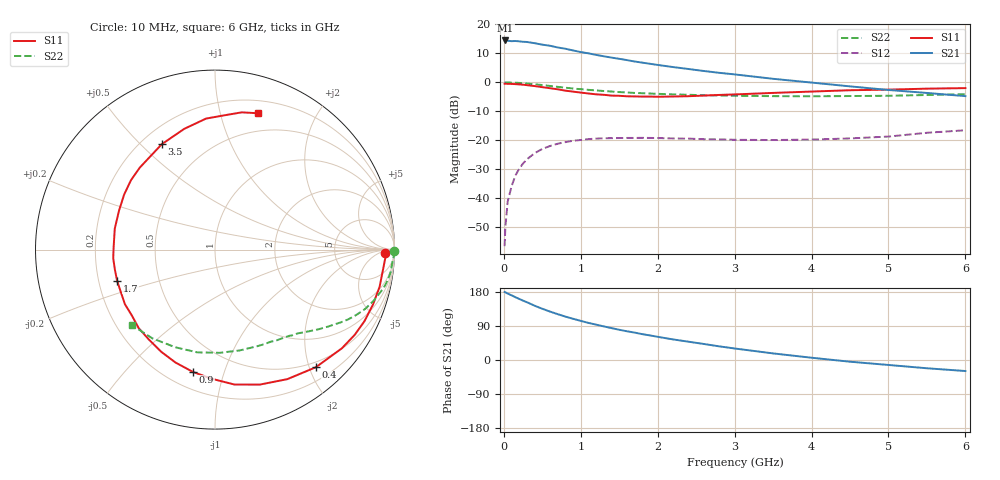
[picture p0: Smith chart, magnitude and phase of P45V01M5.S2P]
! SIEMENS Small Signal Semiconductors
! BFP182
! Si NPN RF Bipolar Junction Transistor in SOT143
! VCE = 5 V  IC = 1.5 mA
! Common Emitter S-Parameters:  March  1996
# GHz  S  MA  R  50
!  f  S11  S21  S12  S22
! GHz  MAG  ANG  MAG  ANG  MAG  ANG  MAG  ANG
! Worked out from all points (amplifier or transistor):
!   36 points, 10 MHz to 6 GHz, reference 50 ohm
!   highest |S21| = 14.4 dB at 20 MHz (marker M1)
!   |S21| within 3 dB of that: start of sweep to 824.5 MHz
!   unconditionally stable (mu >= 1): 2.428 GHz to end of sweep
!   at 250 MHz: K = 0.11, MSG = 21.0 dB, |S12| = -28.0 dB
!   at 1.4 GHz: K = 0.60, MSG = 13.9 dB, |S12| = -19.2 dB
!   at 6 GHz: K = 1.02, MAG = 5.0 dB, |S12| = -16.5 dB
!   S11 on the Smith chart (normalised r, x): 10 MHz: 32, -13; 400 MHz: 0.41, -2.11; 900 MHz: 0.30, -0.79; 1.7 GHz: 0.28, -0.14; 3.5 GHz: 0.28, +0.58; 6 GHz: 0.32, +1.31
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0.01  0.9477 -1.2  5.166 179.3  0.0015 87.3  0.9987 -0.5
0.02  0.9509 -2.4  5.278 178.7  0.0032 83.7  0.9955 -0.9
0.05  0.9433 -6.4  5.221 175.3  0.0088 87.8  0.9961 -2.4
0.1  0.9402 -12.7  5.129 170.7  0.0161 80.2  0.9891 -4.8
0.15  0.9319 -19.2  5.167 165.8  0.0248 77.6  0.9864 -7.3
0.2  0.9233 -25.6  5.095 161.1  0.0324 74.6  0.9787 -9.6
0.3  0.8955 -37.9  4.971 152.5  0.0472 68.0  0.9548 -14.0
0.4  0.8633 -49.4  4.734 143.3  0.0601 60.6  0.9271 -18.1
0.5  0.8267 -60.8  4.469 135.2  0.0712 54.4  0.899 -21.6
0.6  0.7926 -71.6  4.275 127.8  0.0799 49.2  0.8677 -24.8
0.8  0.72 -91.4  3.798 114.5  0.0934 39.3  0.809 -30.1
0.9  0.6926 -100.2  3.553 108.8  0.0984 35.5  0.7832 -32.2
1.1  0.6432 -117.8  3.164 97.9  0.1052 28.8  0.7429 -36.0
1.4  0.5912 -141.5  2.672 84.2  0.1093 20.7  0.6949 -40.9
1.7  0.5723 -162.4  2.29 72.3  0.1102 15.3  0.6571 -45.2
1.9  0.5691 -175.1  2.09 64.8  0.1102 12.4  0.6422 -48.1
2.2  0.5705 168.2  1.836 54.3  0.1079 9.7  0.6211 -52.5
2.8  0.6071 140.5  1.461 36.0  0.104 7.1  0.5941 -62.4
3.5  0.6578 116.8  1.152 17.4  0.1014 8.4  0.5784 -76.2
4.5  0.7317 93.9  0.853 -4.5  0.1081 13.8  0.581 -99.8
5.5  0.779 79.0  0.657 -21.8  0.1352 17.6  0.6054 -125.3
6  0.7962 72.6  0.579 -29.1  0.1494 15.2  0.6256 -138.0
